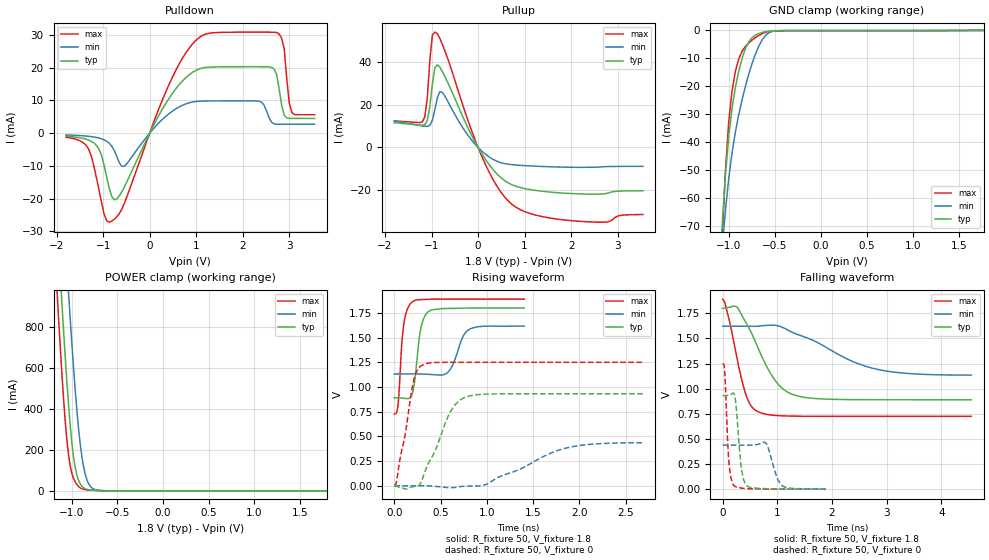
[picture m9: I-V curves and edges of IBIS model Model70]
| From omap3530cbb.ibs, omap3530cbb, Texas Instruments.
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| Model based on original model for BQ0226CS_7LM
|   Sub model BQ0226CS_7LM_PU_ON_1P8
[model]   Model70
|[Input Load]   PU
|[Output Drive]
|Voltage   1.8V
|Mode   I/O
Model_type   I/O
Polarity   Non-Inverting
Enable   Active-Low
Vinl =  0.63
Vinh =  1.17
Cref =  15.0000pF
Rref =  100.0000M
Vref =  0V
Vmeas =  0.9
C_comp   0.742316p   0.619633p   0.9008309p
[Model Spec]
Vinl   0.63   0.567   0.6615
Vinh   1.17   1.053   1.2285
[Temperature Range]   25   125   -40
[Voltage Range]   1.8   1.62   1.89
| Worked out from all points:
|   slope of the pulldown table from 0 to 0.27 V, typ, clamps not added: 37.2 ohm
|   slope of the pullup table from 0 to 0.27 V, typ, clamps not added: 30.1 ohm
|   GND clamp passes 1 mA (typ) near -0.66 V on its own axis
|   POWER clamp passes 1 mA (typ) near -0.62 V on its own axis
|   rising waveform, R_fixture 50, V_fixture 1.8: 20-80 % time 70.6ps typ, 113ps min, 54.4ps max; typ from 0.89 V to 1.8 V
|   rising waveform, R_fixture 50, V_fixture 0: 20-80 % time 255ps typ, 611ps min, 137ps max; typ from 0.002 V to 0.932 V
|   falling waveform, R_fixture 50, V_fixture 1.8: 20-80 % time 508ps typ, 1.11ns min, 284ps max; typ from 1.8 V to 0.89 V
|   falling waveform, R_fixture 50, V_fixture 0: 20-80 % time 89.6ps typ, 150ps min, 64.6ps max; typ from 0.932 V to 0.002 V
[POWER_clamp]
-1.8V     6.299A     6.506A     6.196A
-1.164V   1.344A     1.893A     994.1mA
-1.127V   1.063A     1.63A      711.8mA
-1.109V   925.8mA    1.498A     579.2mA
-1.073V   661.6mA    1.236A     346.9mA
-1.036V   426.8mA    976.9mA    179.1mA
-981.8mV  170.9mA    611.1mA    62.74mA
-909.1mV  36.27mA    236.5mA    15.49mA
-872.7mV  16.52mA    123mA      7.916mA
-836.4mV  7.94mA     57.24mA    5.192mA
-727.3mV  2.334mA    4.383mA    2.32mA
1.8V      4.504nA    2.553nA    7.519nA
[Pulldown]
-1.8V     -923.4uA   -546.6uA   -1.251mA
-1.364V   -1.871mA   -894.2uA   -3.779mA
-1.145V   -3.734mA   -1.313mA   -13.56mA
-818.2mV  -19.23mA   -3.924mA   -26.88mA
-545.5mV  -16.45mA   -10.11mA   -21.46mA
600mV     14.23mA    7.738mA    20.24mA
1.364V    20.2mA     9.834mA    30.64mA
2.618V    20.12mA    3.366mA    30.81mA
2.782V    13.57mA    2.716mA    30.25mA
2.891V    5.528mA    2.714mA    25.85mA
3.055V    4.494mA    2.712mA    6.327mA
3.545V    4.488mA    2.709mA    5.61mA
[Pullup]
-1.8V     11.56mA    12.44mA    12.38mA
-1.145V   10.65mA    9.865mA    14.2mA
-1.091V   12.57mA    9.798mA    23mA
-1.036V   19.01mA    10.29mA    40.58mA
-981.8mV  29.64mA    12.69mA    52.61mA
-927.3mV  37.42mA    17.78mA    54mA
-818.2mV  37.48mA    26.16mA    50.92mA
-763.6mV  35.38mA    25.7mA     48.06mA
54.55mV   -2.036mA   -1.184mA   -2.863mA
709.1mV   -17.28mA   -8.025mA   -26.29mA
2.073V    -21.67mA   -9.32mA    -34.42mA
3.545V    -20.3mA    -8.865mA   -31.43mA
[GND_clamp]
-1.8V     -645.6mA   -500mA     -849.8mA
-1.073V   -71.06mA   -78.88mA   -76.39mA
-1.036V   -52.52mA   -64.92mA   -51.19mA
-1V       -38.11mA   -53.22mA   -32.95mA
-963.6mV  -27.87mA   -43.86mA   -21.7mA
-927.3mV  -20.42mA   -36.37mA   -14.67mA
-890.9mV  -14.61mA   -30.16mA   -10.19mA
-818.2mV  -6.48mA    -19.91mA   -5.73mA
-709.1mV  -1.688mA   -8.413mA   -2.581mA
-600mV    -465.2uA   -1.748mA   -693.5uA
-490.9mV  -144.7uA   -181.9uA   -187.8uA
1.764V    -5.55uA    13.96uA    -26.17uA
[Ramp]
dV/dt_f  0.5575875/0.5188285n  0.2993806/1.159323n   0.7141007/0.2905902n
dV/dt_r  0.5792629/0.2627681n  0.2756467/0.6399178n  0.7758393/0.1410512n
R_load = 50
[Rising Waveform]
R_fixture = 50
V_fixture = 1.8
V_fixture_min = 1.62
V_fixture_max = 1.89
0s        890.2mV    1.132V     725.7mV
42ps      890.3mV    1.132V     835.1mV
82ps      888.4mV    1.132V     1.451V
104ps     886.4mV    1.133V     1.644V
188ps     915.3mV    1.133V     1.857V
280ps     1.564V     1.132V     1.884V
358ps     1.755V     1.129V     1.888V
586ps     1.795V     1.155V     1.89V
826ps     1.799V     1.591V     1.89V
1.404ns   1.8V       1.617V     1.89V
[Rising Waveform]
R_fixture = 50
V_fixture = 0
V_fixture_min = 0
V_fixture_max = 0
0s        2.01mV     1.18mV     2.476mV
24ps      -4.996mV   1.18mV     45.42mV
212ps     -6.218mV   1.415mV    1.077V
274ps     12.23mV    1.433mV    1.204V
314ps     98.62mV    1.338mV    1.227V
600ps     740.3mV    -19.07mV   1.25V
770ps     898.5mV    -2.216mV   1.25V
998ps     928.6mV    16.67mV    1.251V
1.856ns   932.2mV    382.8mV    1.251V
2.686ns   932.3mV    436.3mV    1.251V
[Falling Waveform]
R_fixture = 50
V_fixture = 1.8
V_fixture_min = 1.62
V_fixture_max = 1.89
0s        1.8V       1.62V      1.89V
130ps     1.809V     1.62V      1.659V
256ps     1.813V     1.62V      1.321V
412ps     1.669V     1.62V      964mV
524ps     1.557V     1.62V      826.6mV
664ps     1.384V     1.622V     767.6mV
970ps     1.075V     1.629V     734mV
1.368ns   928.1mV    1.539V     726.9mV
2.812ns   890.5mV    1.194V     725.7mV
4.548ns   890.2mV    1.135V     725.7mV
[Falling Waveform]
R_fixture = 50
V_fixture = 0
V_fixture_min = 0
V_fixture_max = 0
0s        932.3mV    439.5mV    1.251V
40ps      931.7mV    439.6mV    1.151V
116ps     935.9mV    439.4mV    264.4mV
208ps     952.1mV    439.2mV    38.25mV
242ps     849.6mV    439.1mV    25.45mV
346ps     195.5mV    439.1mV    12.72mV
446ps     35.51mV    439.2mV    7.207mV
780ps     6.927mV    467.3mV    3.568mV
1.124ns   3.782mV    25.67mV    2.674mV
1.89ns    2.256mV    4.429mV    2.483mV
